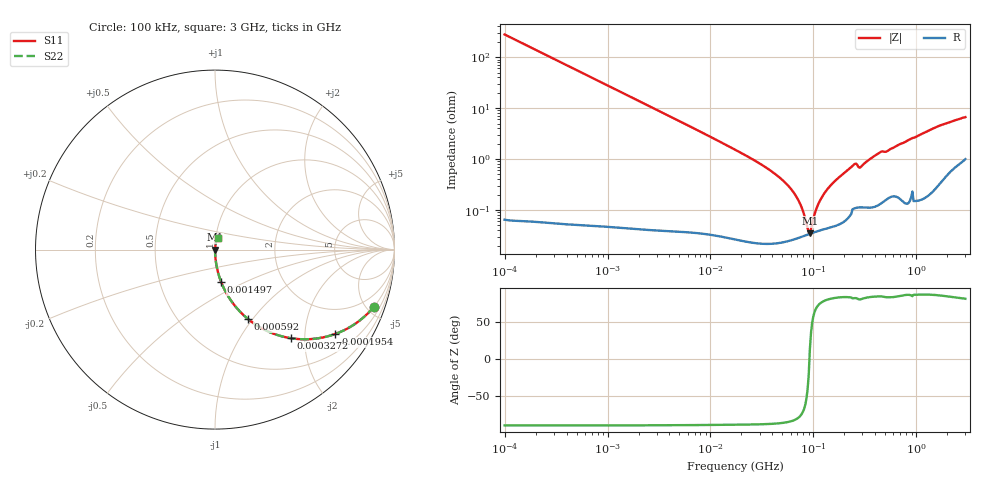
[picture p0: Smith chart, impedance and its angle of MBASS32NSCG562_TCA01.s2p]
! MBASS32NSCG562_TCA01  S-PARAMETER MODEL  ( Standard Model )
! Model Generated by TAIYO YUDEN Corporation (https://www.yuden.co.jp/en/)
! Version 1.0
! TAIYO YUDEN Control No. 250312
! Copyright(c) 2025 TAIYO YUDEN CO.,LTD. All Rights Reserved.
! Product Description (link to TY-COMPAS)
! https://ds.yuden.co.jp/TYCOMPAS/or/detail?pn=MBASS32NSCG562JTCA01&u=M
! Products Name : Multilayer Ceramic Capacitors
! Characteristics :
!  Capacitance : 5600 [pF] , Rated Voltage : 630 [V] , TCC : CG / C0G
!  Case Size : 3.2 x 2.5 / 0.126 x 0.098 [mm/inch] , Thickness : 1.9 / 0.075 [mm/inch]
!  (Conditions: Temperature = 25 [degC] , DC Bias Voltage = 0 [V])
! External Node Assignments :
!  1  o---| |---o  2
! GND o---------o GND
! Frequency Range : 0.1MHz  -  3000MHz  [ 401 STEP ]
# MHZ S RI R 50
! Freq[MHz].  S11 Real  S11 Imag  S21 Real  S21 Imag  S12 Real  S12 Imag  S22 Real  S22 Imag
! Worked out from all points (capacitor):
!   401 points, 100 kHz to 3 GHz, reference 50 ohm
!   read as one part in series: C = 5.71 nF near 105.3 kHz
!   lowest |Z| = 35.2 mohm at 92.49 MHz (marker M1)
!   series resonance near 91.6 MHz, so ESL is about 530 pH
!   S11 on the Smith chart (normalised r, x): 100 kHz: 1.00, -5.58; 195.4 kHz: 1.00, -2.86; 327.2 kHz: 1.00, -1.71; 592 kHz: 1.00, -0.94; 1.497 MHz: 1.00, -0.37; 3 GHz: 1.02, +0.13
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0.1  0.8861 -0.3176  0.1139 0.3176  0.1139 0.3176  0.8861 -0.3176
0.19544  0.6711 -0.4696  0.3289 0.4696  0.3289 0.4696  0.6711 -0.4696
0.327242  0.4211 -0.4934  0.5789 0.4934  0.5789 0.4934  0.4211 -0.4934
0.562235  0.198 -0.398  0.802 0.398  0.802 0.398  0.198 -0.398
0.591975  0.1822 -0.3855  0.8178 0.3855  0.8178 0.3855  0.1822 -0.3855
1.497078  0.034 -0.18  0.966 0.18  0.966 0.18  0.034 -0.18
3.161081  0.00811 -0.0875  0.9919 0.0875  0.9919 0.0875  0.00811 -0.0875
17.7727  0.000485 -0.0149  0.9995 0.0149  0.9995 0.0149  0.000485 -0.0149
36.57227  0.000257 -0.00636  0.9997 0.00636  0.9997 0.00636  0.000257 -0.00636
56.67997  0.000255 -0.00303  0.9997 0.00303  0.9997 0.00303  0.000255 -0.00303
71.47675  0.000286 -0.00154  0.9997 0.00154  0.9997 0.00154  0.000286 -0.00154
87.84301  0.00033 -0.000288  0.9997 0.000288  0.9997 0.000288  0.00033 -0.000288
92.48959  0.000343 8.12e-05  0.9997 -8.12e-05  0.9997 -8.12e-05  0.000343 8.12e-05
97.38194  0.000356 0.000411  0.9996 -0.000411  0.9996 -0.000411  0.000356 0.000411
116.6348  0.000403 0.00152  0.9996 -0.00152  0.9996 -0.00152  0.000403 0.00152
163.0551  0.000502 0.00373  0.9995 -0.00373  0.9995 -0.00373  0.000502 0.00373
246.2744  0.00112 0.00762  0.9989 -0.00762  0.9989 -0.00762  0.00112 0.00762
287.4592  0.00118 0.00682  0.9988 -0.00682  0.9988 -0.00682  0.00118 0.00682
434.1712  0.00144 0.0132  0.9986 -0.0132  0.9986 -0.0132  0.00144 0.0132
547.5153  0.00198 0.0151  0.998 -0.0151  0.998 -0.0151  0.00198 0.0151
1575.075  0.00458 0.0425  0.9954 -0.0425  0.9954 -0.0425  0.00458 0.0425
3000  0.0141 0.0643  0.9859 -0.0643  0.9859 -0.0643  0.0141 0.0643
